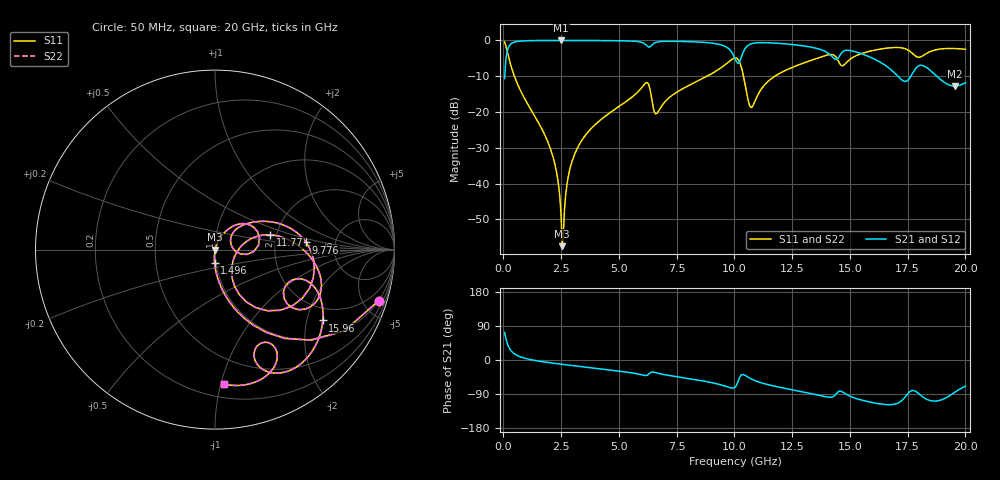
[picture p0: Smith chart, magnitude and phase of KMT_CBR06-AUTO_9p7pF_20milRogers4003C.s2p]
! Data measured by Modelithics Inc. support@modelithics.com 813-866-6335
! KEMET CBR06-AUTO 9.7pF, Pad Width= 0.851mm, Pad Length= 0.64mm, Pad Gap= 0.62mm, 20mil Rogers 4003C substrate Data, January 2022
# hz S ma R 50
! 2 Port Network Data from SP1.SP block
! freq  magS11  angS11  magS21  angS21  magS12  angS12  magS22  angS22
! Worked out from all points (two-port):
!   401 points, 50 MHz to 20 GHz, reference 50 ohm
!   highest |S21| = -0.01 dB at 2.494 GHz (marker M1); lowest = -12.8 dB at 19.55 GHz (marker M2)
!   |S21| within 3 dB of the highest: 165.5 MHz to 9.85 GHz (9.685 GHz wide, 193 % of centre); 10.4 GHz to 13.91 GHz (3.507 GHz wide, 28.9 % of centre)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
!   lowest |S11| = -57.5 dB at 2.544 GHz (marker M3), VSWR 1.00, Z = 50.1 - j0.11 ohm
!   |S11| at or under -10 dB: 473.2 MHz to 8.812 GHz (8.339 GHz wide, 180 % of centre); 10.39 GHz to 11.75 GHz (1.358 GHz wide, 12.3 % of centre)
!   |S22| runs from -57.5 to -0.4 dB; largest |S21 - S12| = 0
!   S11 on the Smith chart (normalised r, x): 50 MHz: 0.98, -6.43; 1.496 GHz: 0.98, -0.14; 9.776 GHz: 3.04, +0.33; 11.77 GHz: 1.85, +0.34; 15.96 GHz: 1.53, -2.51; 20 GHz: 0.30, -1.02
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5e7  0.9559 -17.3  0.2934 72.7  0.2934 72.7  0.9559 -17.3
4.49e8  0.3322 -72.5  0.9426 17.4  0.9426 17.4  0.3322 -72.5
1.496375e9  0.07287 -91.9  0.9965 -2.6  0.9965 -2.6  0.07287 -91.9
2.194625e9  0.02057 -96.2  0.9988 -8.7  0.9988 -8.7  0.02057 -96.2
2.493875e9  0.003704 -86.0  0.9989 -11.0  0.9989 -11.0  0.003704 -86.0
2.54375e9  0.001337 -54.9  0.9989 -11.4  0.9989 -11.4  0.001337 -54.9
2.892875e9  0.01674 72.5  0.9987 -14.0  0.9987 -14.0  0.01674 72.5
3.391625e9  0.04014 70.8  0.9979 -17.5  0.9979 -17.5  0.04014 70.8
6.13475e9  0.25 29.3  0.8871 -40.9  0.8871 -40.9  0.25 29.3
6.73325e9  0.1058 34.4  0.9587 -35.6  0.9587 -35.6  0.1058 34.4
9.775625e9  0.5092 4.5  0.7537 -72.6  0.7537 -72.6  0.5092 4.5
1.0025e10  0.5701 -16.4  0.5592 -71.8  0.5592 -71.8  0.5701 -16.4
1.027438e10  0.4479 -49.5  0.5545 -41.1  0.5545 -41.1  0.4479 -49.5
1.072325e10  0.1154 -21.8  0.8963 -49.8  0.8963 -49.8  0.1154 -21.8
1.177062e10  0.3194 14.9  0.9164 -69.5  0.9164 -69.5  0.3194 14.9
1.336662e10  0.5327 -4.5  0.7996 -89.3  0.7996 -89.3  0.5327 -4.5
1.46135e10  0.4487 -31.8  0.6528 -82.4  0.6528 -82.4  0.4487 -31.8
1.596012e10  0.719 -33.3  0.5687 -112.1  0.5687 -112.1  0.719 -33.3
1.670825e10  0.7867 -47.5  0.407 -117.9  0.407 -117.9  0.7867 -47.5
1.770575e10  0.6589 -70.1  0.3443 -80.5  0.3443 -80.5  0.6589 -70.1
1.955112e10  0.77 -79.0  0.2303 -84.7  0.2303 -84.7  0.77 -79.0
2e10  0.7515 -86.2  0.2563 -69.2  0.2563 -69.2  0.7515 -86.2
